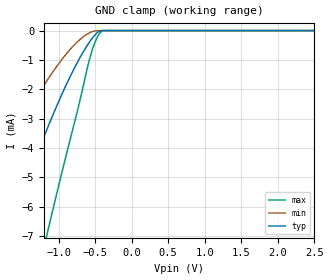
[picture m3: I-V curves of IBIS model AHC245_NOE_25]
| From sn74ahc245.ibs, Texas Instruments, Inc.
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[Model]   AHC245_NOE_25
Model_type  Input
Vinl = 0.5
Vinh = 1.7
| variable   typ   min   max
C_comp   0.74pF   0.68pF   0.80pF
[Temperature Range]   40   100   -40
| Ambient temperature   25   85   -40
[Voltage range]   2.5   2.3   2.7
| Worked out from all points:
|   GND clamp passes 1 mA (typ) near -0.73 V on its own axis
[GND Clamp]
| AHC245_NOE_25
|   Voltage   I(typ)   I(min)   I(max)
-2.5V     -12.87mA   -7.885mA   -22.93mA
-2.275V   -11.15mA   -6.751mA   -20.07mA
-1.695V   -6.911mA   -3.966mA   -12.99mA
-1.655V   -6.631mA   -3.784mA   -12.52mA
-1.145V   -3.273mA   -1.649mA   -6.795mA
-835mV    -1.53mA    -620.6uA   -3.643mA
-595mV    -455.3uA   -100.6uA   -1.148mA
-545mV    -278.4uA   -42.97uA   -699uA
-490mV    -115.5uA   -9.938uA   -324.4uA
-440mV    -19.96uA   -5.07uA    -101.3uA
-390mV    -45.18nA   -2.497uA   -3.537uA
2.5V      15.78pA    59.61pA    12.5pA
